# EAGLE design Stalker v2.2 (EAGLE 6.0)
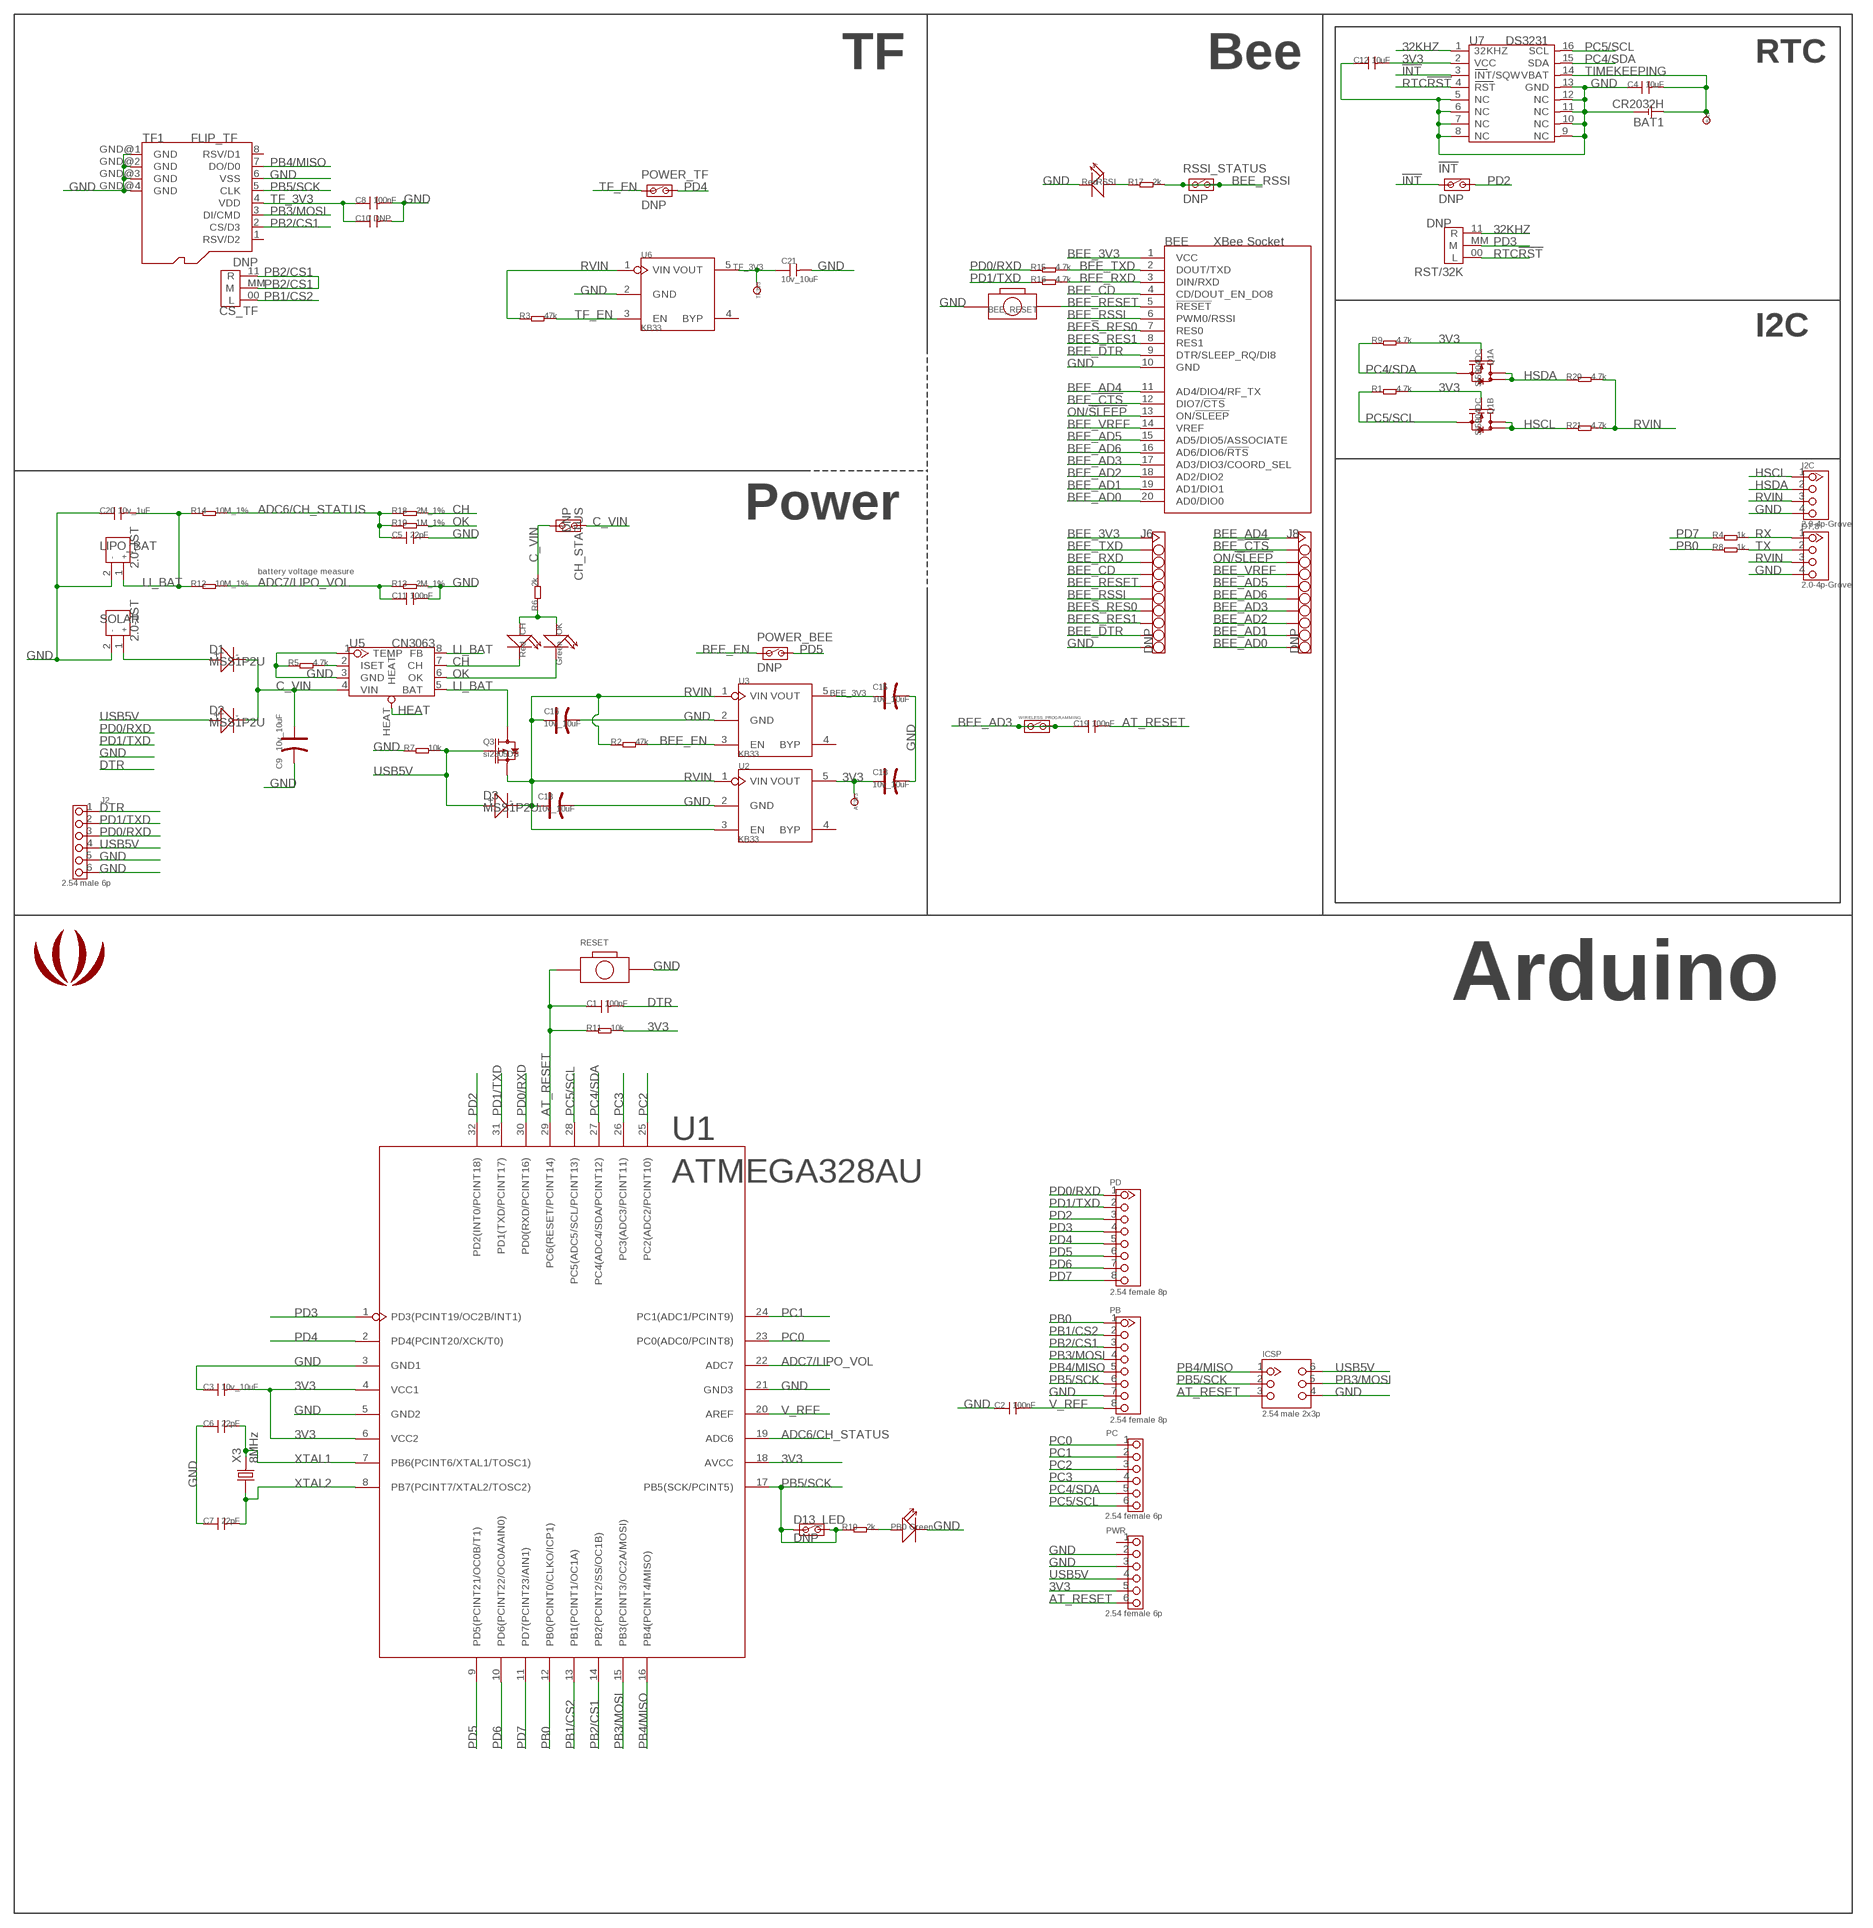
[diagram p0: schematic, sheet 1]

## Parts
!INT  DNP  JP_SW  [JP_SW]
AT3V3  DNP  TEST_POINT_SIZE_3030  [TP_3535]
BAT  DNP  TEST_POINT_SIZE_3030  [TP_3535]
BAT1  CR2032H  [CR2032H]
BEE  XBee Socket  BEEO  [BEE]
BEE_RESET  3.8x6.1 button  BOTTON_1_SMD  [BOTTON_1]
C1  100nF  C-0603  [0603]
C2  100nF  C-0603  [0603]
C3  10v_10uF  C-0805  [0805]
C4  10uF  C-0805  [0805]
C5  22pF  C-0603  [0603]
C6  22pF  C-0603  [0603]
C7  22pF  C-0603  [0603]
C8  100nF  C-0603  [0603]
C9  10v_10uF  CAP-AVX-A  [AVX-A]
C10  DNP  C-0603  [0603]
C11  100nF  C-0603  [0603]
C12  10uF  C-0805  [0805]
C13  10v_10uF  CAP-AVX-A  [AVX-A]
C15  10v_10uF  CAP-AVX-A  [AVX-A]
C16  10v_10uF  CAP-AVX-A  [AVX-A]
C18  10v_10uF  CAP-AVX-A  [AVX-A]
C19  100nF  C-0603  [0603]
C20  10v_1uF  C-0805  [0805]
C21  10v_10uF  C-0805  [0805]
CH  Red  007-LED0603  [D0603]
CH_STATUS  DNP  JP_SW  [JP_SW]
CS_TF  DNP  JUMPER  [JUMPER]
D1  MSS1P2U  010-DMSS1P2U  [D1005]
D2  MSS1P2U  010-DMSS1P2U  [D1005]
D3  MSS1P2U  010-DMSS1P2U  [D1005]
D7,8  2.0-4p-Grove  TWIG-4P-2.0-2.0  [4P-2.0]
D13_LED  DNP  JP_SW  [JP_SW]
I2C  2.0-4p-Grove  TWIG-4P-2.0-2.0  [4P-2.0]
ICSP  2.54 male 2x3p  HEADER-2X3P-2.54  [2X3P-2.54-LEADED]
J2  2.54 male 6p  HEADER-6P-LEADED-2.54  [6P-2.54-LEADED]
J6  DNP  HEADER_1X10DD  [HEADER_1X10]
J8  DNP  HEADER_1X10DD  [HEADER_1X10]
LIPO_BAT  2.0-JST  JACK-JST-2P-PW'2.0'  [JST-2.0]
LOGO1  LOGO  [LOGO_RO]
OK  Green  007-LED0603  [D0603]
PB  2.54 female 8p  HEADER-8P-2.54-LEADED  [8P-2.54-LEADED]
PB0  Green  007-LED0603  [D0603]
PC  2.54 female 6p  HEADER-6P-LEADED-2.54  [6P-2.54-LEADED]
PD  2.54 female 8p  HEADER-8P-2.54-LEADED  [8P-2.54-LEADED]
POWER_BEE  DNP  JP_SW  [JP_SW]
POWER_TF  DNP  JP_SW  [JP_SW]
PWR  2.54 female 6p  HEADER-6P-LEADED-2.54  [6P-2.54-LEADED]
Q1  Si5904DC  010-DUAL-N-MOSFET_1206-8  [1206-8]
Q3  si2305DS  010-P-MOSFETSOT23  [SOT23]
R1  4.7k  005-R0603  [0603@1]
R2  47k  005-R0603  [0603@1]
R3  47k  005-R0603  [0603@1]
R4  1k  005-R0603  [0603@1]
R5  4.7k  005-R0603  [0603@1]
R6  2k  005-R0603  [0603@1]
R7  10k  005-R0603  [0603@1]
R8  1k  005-R0603  [0603@1]
R9  4.7k  005-R0603  [0603@1]
R10  2k  005-R0603  [0603@1]
R11  10k  005-R0603  [0603@1]
R12  10M_1%  005-R0603  [0603@1]
R13  2M_1%  005-R0603  [0603@1]
R14  10M_1%  005-R0603  [0603@1]
R15  4.7k  005-R0603  [0603@1]
R16  4.7k  005-R0603  [0603@1]
R17  2k  005-R0603  [0603@1]
R18  2M_1%  005-R0603  [0603@1]
R19  1M_1%  005-R0603  [0603@1]
R20  4.7k  005-R0603  [0603@1]
R21  4.7k  005-R0603  [0603@1]
RESET  3.8x6.1 button  BOTTON_1_SMD  [BOTTON_1]
RSSI  Red  007-LED0603  [D0603]
RSSI_STATUS  DNP  JP_SW  [JP_SW]
RST/32K  DNP  JUMPER  [JUMPER]
SOLAR  2.0-JST  JACK-JST-2P-PW'2.0'  [JST-2.0]
TF1  FLIP_TF  [FLIP_TF]
TF3V3  DNP  TEST_POINT_SIZE_3030  [TP_3535]
U1  ATMEGA328AU  ATMEGA168-20AU  [ATMEGA168-20AU]
U2  KB33  MIC5025_X.X  [SOT23-5]
U3  KB33  MIC5025_X.X  [SOT23-5]
U5  CN3063  CN3083  [SOP8]
U6  KB33  MIC5025_X.X  [SOT23-5]
U7  DS3231  [SO16-W]
WIRELESS_PROGRAMMING  DNP  JP_SW  [JP_SW]
X3  8MHz  011-CRYSTALHC49S  [HC49/S]

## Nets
3V3: AT3V3.T C3.2 C12.2 C13.+ PWR.5 Q1.2(A:G) Q1.4(B:G) R1.2 R9.2 R11.2 U1.4(VCC1) U1.6(VCC2) U1.18(AVCC) U2.5(VOUT) U7.2(VCC)
32KHZ: RST/32K.11(R) U7.1(32KHZ)
!INT: !INT.1 U7.3(INT/SQW)
ADC6/CH_STATUS: C5.1 R14.2 R18.1 R19.1 U1.19(ADC6)
ADC7/LIPO_VOL: C11.1 R12.2 R13.1 U1.22(ADC7)
AT_RESET: C1.1 C19.2 ICSP.3 PWR.6 R11.1 RESET.1 U1.29(PC6(RESET/PCINT14))
BEE_3V3: BEE.1(VCC) C15.+ J6.1 U3.5(VOUT)
BEE_!CTS: BEE.12(DIO7/!CTS) J8.2
BEE_AD0: BEE.20(AD0/DIO0) J8.10
BEE_AD1: BEE.19(AD1/DIO1) J8.9
BEE_AD2: BEE.18(AD2/DIO2) J8.8
BEE_AD3: BEE.17(AD3/DIO3/COORD_SEL) C19.1 J8.7 WIRELESS_PROGRAMMING.1 WIRELESS_PROGRAMMING.2
BEE_AD4: BEE.11(AD4/DIO4/RF_TX) J8.1
BEE_AD5: BEE.15(AD5/DIO5/ASSOCIATE) J8.5
BEE_AD6: BEE.16(AD6/DIO6/!RTS) J8.6
BEE_CD: BEE.4(CD/DOUT_EN_DO8) J6.4
BEE_DTR: BEE.9(DTR/SLEEP_RQ/DI8) J6.9
BEE_EN: POWER_BEE.1 R2.2 U3.3(EN)
BEE_RESET: BEE.5(!RESET) BEE_RESET.P$2 J6.5
BEE_RSSI: BEE.6(PWM0/RSSI) J6.6 R17.2 RSSI_STATUS.1 RSSI_STATUS.2
BEE_RXD: BEE.3(DIN/RXD) J6.3 R16.2
BEE_TXD: BEE.2(DOUT/TXD) J6.2 R15.2
BEE_VREF: BEE.14(VREF) J8.4
BEES_RES0: BEE.7(RES0) J6.7
BEES_RES1: BEE.8(RES1) J6.8
C_VIN: C9.+ CH_STATUS.1 CH_STATUS.2 D1.- D2.- R6.2 U5.4(VIN)
CH: CH.- R18.2 U5.7(CH)
DTR: C1.2 J2.1
GND: BAT1.- BEE.10(GND) BEE_RESET.1 C2.1 C3.1 C4.1 C5.2 C6.1 C7.1 C8.2 C9.- C10.2 C11.2 C12.1 C13.- C15.- C16.- C18.- C20.1 C21.2 D7,8.4 I2C.4 ICSP.4 J2.5 J2.6 J6.10 LIPO_BAT.2 PB0.- PB.7 PWR.2 PWR.3 R5.1 R7.1 R13.2 RESET.P$2 RSSI.- SOLAR.2 TF1.6(VSS) TF1.GND@1(GND) TF1.GND@2(GND) TF1.GND@3(GND) TF1.GND@4(GND) U1.3(GND1) U1.5(GND2) U1.21(GND3) U2.2(GND) U3.2(GND) U5.1(TEMP) U5.3(GND) U6.2(GND) U7.5(NC) U7.6(NC) U7.7(NC) U7.8(NC) U7.9(NC) U7.10(NC) U7.11(NC) U7.12(NC) U7.13(GND)
HEAT: U5.HEAT
HSCL: I2C.1 Q1.5(B:D) Q1.6(B:D) R21.1
HSDA: I2C.2 Q1.7(A:D) Q1.8(A:D) R20.1
LI_BAT: C20.2 LIPO_BAT.1 Q3.3(D) R12.1 R14.1 U5.5(BAT) U5.8(FB)
N$1: PB0.+ R10.2
N$3: D1.+ SOLAR.1
N$5: R5.2 U5.2(ISET)
N$6: R17.1 RSSI.+
N$8: CH.+ OK.+ R6.1
OK: OK.- R19.2 U5.6(OK)
ON/!SLEEP: BEE.13(ON/!SLEEP) J8.3
PB0: PB.1 R8.1 U1.12(PB0(PCINT0/CLKO/ICP1))
PB1/CS2: CS_TF.00(L) PB.2 U1.13(PB1(PCINT1/OC1A))
PB2/CS1: CS_TF.11(R) CS_TF.MM(M) PB.3 TF1.2(CS/D3) U1.14(PB2(PCINT2/SS/OC1B))
PB3/MOSI: ICSP.5 PB.4 TF1.3(DI/CMD) U1.15(PB3(PCINT3/OC2A/MOSI))
PB4/MISO: ICSP.1 PB.5 TF1.7(DO/D0) U1.16(PB4(PCINT4/MISO))
PB5/SCK: D13_LED.1 D13_LED.2 ICSP.2 PB.6 R10.1 TF1.5(CLK) U1.17(PB5(SCK/PCINT5))
PC0: PC.1 U1.23(PC0(ADC0/PCINT8))
PC1: PC.2 U1.24(PC1(ADC1/PCINT9))
PC2: PC.3 U1.25(PC2(ADC2/PCINT10))
PC3: PC.4 U1.26(PC3(ADC3/PCINT11))
PC4/SDA: PC.5 Q1.1(A:S) R9.1 U1.27(PC4(ADC4/SDA/PCINT12)) U7.15(SDA)
PC5/SCL: PC.6 Q1.3(B:S) R1.1 U1.28(PC5(ADC5/SCL/PCINT13)) U7.16(SCL)
PD0/RXD: J2.3 PD.1 R15.1 U1.30(PD0(RXD/PCINT16))
PD1/TXD: J2.2 PD.2 R16.1 U1.31(PD1(TXD/PCINT17))
PD2: !INT.2 PD.3 U1.32(PD2(INT0/PCINT18))
PD3: PD.4 RST/32K.MM(M) U1.1(PD3(PCINT19/OC2B/INT1))
PD4: PD.5 POWER_TF.2 U1.2(PD4(PCINT20/XCK/T0))
PD5: PD.6 POWER_BEE.2 U1.9(PD5(PCINT21/OC0B/T1))
PD6: PD.7 U1.10(PD6(PCINT22/OC0A/AIN0))
PD7: PD.8 R4.1 U1.11(PD7(PCINT23/AIN1))
RTC!RST: RST/32K.00(L) U7.4(RST)
RVIN: C16.+ C18.+ D3.- D7,8.3 I2C.3 Q3.2(S) R2.1 R3.1 R20.2 R21.2 U2.1(VIN) U2.3(EN) U3.1(VIN) U6.1(VIN)
RX: D7,8.1 R4.2
TF_3V3: C8.1 C10.1 C21.1 TF1.4(VDD) TF3V3.T U6.5(VOUT)
TF_EN: POWER_TF.1 R3.2 U6.3(EN)
TIMEKEEPING: BAT1.+ BAT.T C4.2 U7.14(VBAT)
TX: D7,8.2 R8.2
USB5V: D2.+ D3.+ ICSP.6 J2.4 PWR.4 Q3.1(G) R7.2
V_REF: C2.2 PB.8 U1.20(AREF)
XTAL1: C6.2 U1.7(PB6(PCINT6/XTAL1/TOSC1)) X3.2
XTAL2: C7.2 U1.8(PB7(PCINT7/XTAL2/TOSC2)) X3.1
Unconnected: PWR.1 TF1.1(RSV/D2) TF1.8(RSV/D1) U2.4(BYP) U3.4(BYP) U6.4(BYP)

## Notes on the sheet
- TF | Bee | RTC
- I2C
- Power
- battery voltage measure
- Arduino

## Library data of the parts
!INT CH_STATUS D13_LED POWER_BEE POWER_TF RSSI_STATUS WIRELESS_PROGRAMMING = CPT_SMD:JP_SW
AT3V3 BAT TF3V3 = For_Test_Albert:TEST_POINT
BAT1 = BAT:CR2032H
BEE = EXT_moudle:BEE
BEE_RESET RESET = CPT_SMD:BOTTON_1
C1-C8 C10-C12 C19-C21 = Discrete:C*: Ceramic Capacitors
C9 C13 C15 C16 C18 = Discrete:CAP*: Electrolytic Capacitors,Tantalum Capacitors and Super Capacitors
CH OK PB0 RSSI = Discrete:007-LED*
CS_TF RST/32K = CPT_SMD:JUMPER
D1-D3 = Discrete:010-D*
D7,8 I2C = Connector:TWIG-4P-2.0
ICSP = Connector:HEADER-2X3P
J2 PC PWR = Connector:HEADER-6P
J6 J8 = CONNECTER:HEADER_1X10
LIPO_BAT SOLAR = Connector:JACK-JST-2P-PW
LOGO1 = logo:LOGO
PB PD = Connector:HEADER-8P
Q1 = Discrete:010-DUAL-N-MOSFET*: Si5902BDC Si5904DC Si5908DC Si5920DC
Q3 = Discrete:010-P-MOSFET*: Si2305DS Si2323CDS
R1-R21 = Discrete:005-R*
TF1 = Holders:FLIP_TF: http://garden.seeedstudio.com/images/e/e4/Flip_TF_Holder.jpg
U1 = IC_SMD:ATMEGA168-20AU
U2 U3 U6 = ICs_v54:MIC5025_X.X
U5 = ICs_v54:CN3083
U7 = IC:DS3231: Extremely Accurate I2C-Integrated RTC/TCXO/Crystal http://pdfserv.maxim-ic.com/en/ds/DS3231.pdf
X3 = Discrete:011-CRYSTAL*: CRYSTAL

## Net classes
0 default: width 0.152 mm, drill 0.305 mm, clearance 0.152 mm

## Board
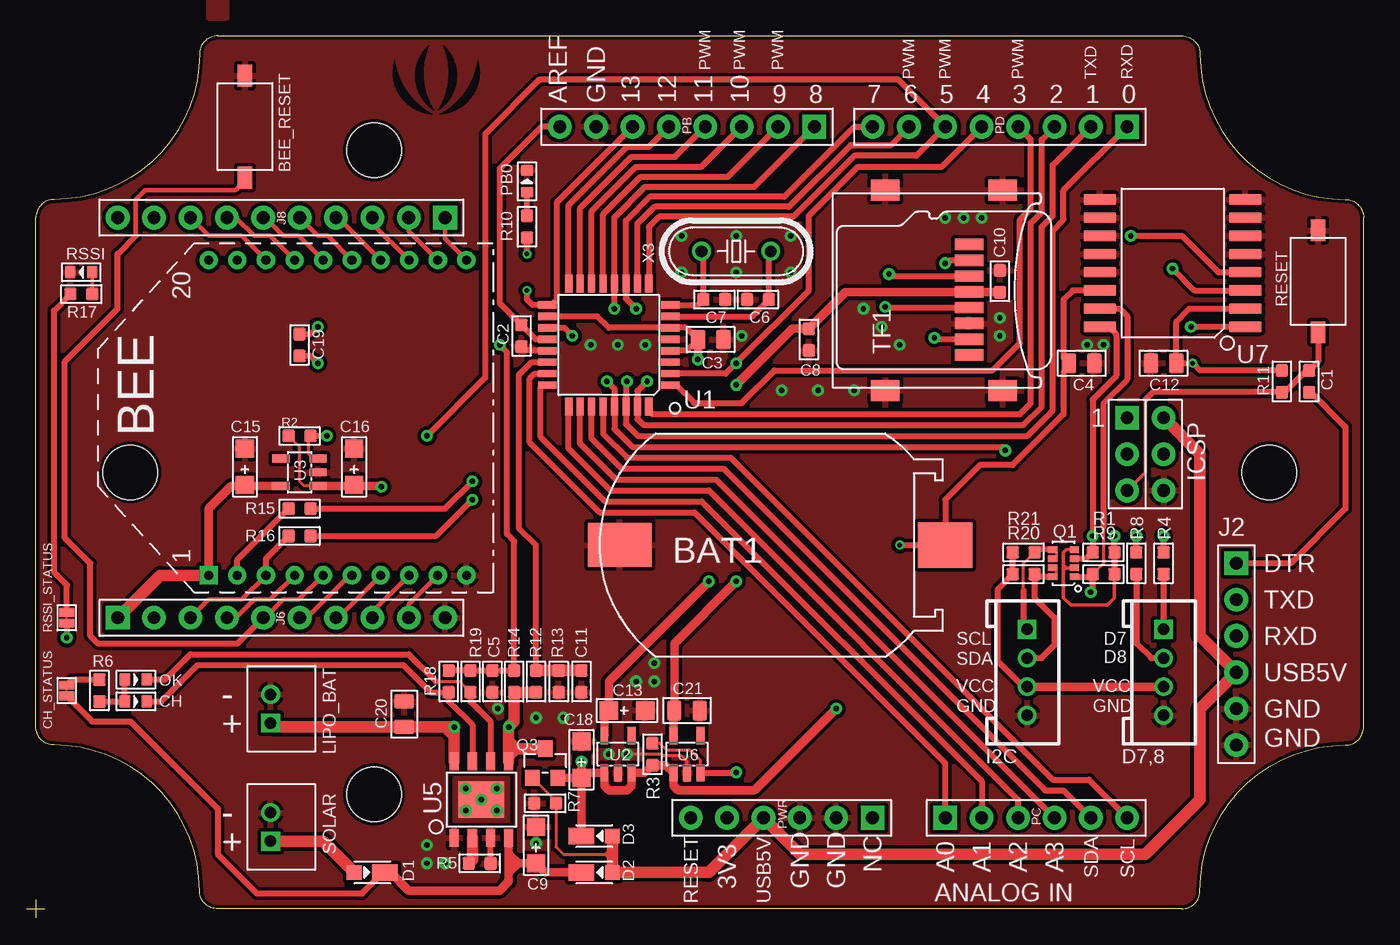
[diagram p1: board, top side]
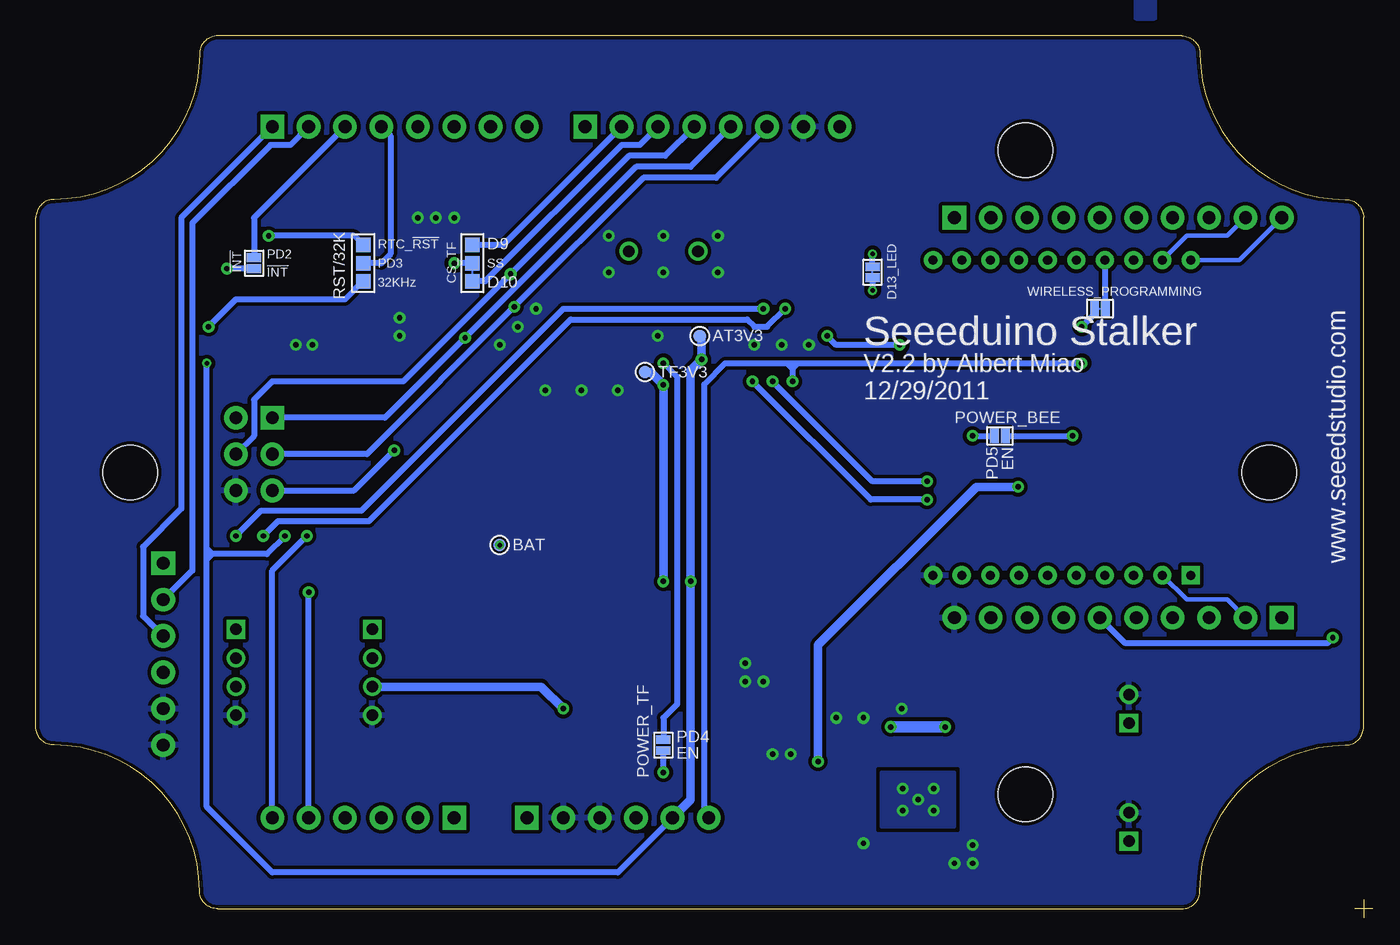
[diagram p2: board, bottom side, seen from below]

Size 92.71 x 60.96 mm. Coordinates in mm from the lower left corner, seen from the top.
Outline: 12.7,60.96 arc90 11.43,59.69 arc-90 1.27,49.53 arc90 0,48.26 0,12.7 arc90 1.27,11.43 arc-90 11.43,1.27 arc90 12.7,0 80.01,0 arc90 81.28,1.27 arc-90 91.44,11.43 arc90 92.71,12.7 92.71,48.26 arc90 91.44,49.53 arc-90 81.28,59.69 arc90 80.01,60.96 12.7,60.96
Copper layers (1*16): Top 0.035mm / dielectric 1.5mm / Bottom 0.035mm
Design rules: minimum track width 6mil, minimum drill 12mil, track to track 6mil, track to pad 6mil, pad to pad 6mil, via to via 6mil, smd to smd 0mil, copper to edge 10mil, drill to drill 10mil, minimum pad ring 10mil, minimum via ring 6mil, stop-mask expansion 2mil, vias tented up to drill 25mil, thermal gap 10mil
Holes 3.81 mm at 23.61,52.98 86.11,30.48 6.61,30.48 23.61,7.98
tRestrict: area 73.7,43.2 to 74.9,48.9; area 83.8,43.2 to 85.1,48.9
Milling: 2 lines

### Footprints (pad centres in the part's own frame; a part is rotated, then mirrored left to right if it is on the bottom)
JP_SW = smd 1.016 x 0.61: 1 0,0.381; 2 0,-0.381
TP_3535 = smd 0.889 x 0.889: T 0,0
CR2032H = smd 3.81 x 3.175: + 12.7,0 | smd 4.445 x 3.048: - -10.033,0
BEE = drill 0.635 pad 1.27 square: 1 -11,0 | drill 0.635 pad 1.27: 2 -11,-2; 3 -11,-4; 4 -11,-6; 5 -11,-8; 6 -11,-10; 7 -11,-12; 8 -11,-14; 9 -11,-16; 10 -11,-18; 11 11,-18; 12 11,-16; 13 11,-14; 14 11,-12; 15 11,-10; 16 11,-8; 17 11,-6; 18 11,-4; 19 11,-2; 20 11,0
BOTTON_1 = smd 1.524 x 1.016: 1 -3.556,0; P$2 3.556,0
0603 = smd 0.889 x 0.889: 1 -0.762,0; 2 0.762,0
0805 = smd 1.016 x 1.397: 1 -0.889,0; 2 0.889,0
AVX-A = smd 1.27 x 1.27: + -1.27,0; - 1.27,0
D0603 = smd 0.762 x 0.889: + -0.762,0; - 0.762,0
JUMPER = smd 1.016 x 1.016: 00 -1.27,0; 11 1.27,0; MM 0,0
D1005 = smd 1.016 x 1.016: + 1.27,0 | smd 1.778 x 1.143: - -0.889,0
4P-2.0 = drill 0.8 pad 1.27 square: 1 -3,0 | drill 0.8 pad 1.27: 2 -1,0; 3 1,0; 4 3,0
2X3P-2.54-LEADED = drill 0.889 pad 1.651 square: 1 -1.27,2.54 | drill 0.889 pad 1.651: 2 -1.27,0; 3 -1.27,-2.54; 4 1.27,-2.54; 5 1.27,0; 6 1.27,2.54
6P-2.54-LEADED = drill 0.889 pad 1.651 square: 1 0,6.35 | drill 0.889 pad 1.651: 2 0,3.81; 3 0,1.27; 4 0,-1.27; 5 0,-3.81; 6 0,-6.35
HEADER_1X10 = drill 0.889 pad 1.651 square: 1 0,11.43 | drill 0.889 pad 1.651: 2 0,8.89; 3 0,6.35; 4 0,3.81; 5 0,1.27; 6 0,-1.27; 7 0,-3.81; 8 0,-6.35; 9 0,-8.89; 10 0,-11.43
JST-2.0 = drill 0.8 pad 1.3 square: 1 -1,0.75 | drill 0.8 pad 1.3: 2 1,0.75
8P-2.54-LEADED = drill 0.889 pad 1.651 square: 1 0,8.89 | drill 0.889 pad 1.651: 2 0,6.35; 3 0,3.81; 4 0,1.27; 5 0,-1.27; 6 0,-3.81; 7 0,-6.35; 8 0,-8.89
1206-8 = smd 0.457 x 0.635: 1 -0.953,-0.762; 2 -0.318,-0.762; 3 0.318,-0.762; 4 0.953,-0.762; 5 0.953,0.762; 6 0.318,0.762; 7 -0.318,0.762; 8 -0.953,0.762
SOT23@1 = smd 1.016 x 1.143: 1 -0.889,-1.016; 2 0.889,-1.016; 3 0,1.016
0603@1 = smd 0.889 x 0.889: 1 -0.762,0; 2 0.762,0
FLIP_TF = smd 0.8 x 2: 1 3.2,0.25; 2 2.1,0.25; 3 1,0.25; 4 -0.1,0.25; 5 -1.2,0.25; 6 -2.3,0.25; 7 -3.4,0.25; 8 -4.5,0.25 | smd 1.45 x 2: GND@1 -7,6.1; GND@2 -7,-2.1; GND@3 7,-2.1; GND@4 7,6.1
ATMEGA168-20AU = smd 1.27 x 0.508: 1 -4.293,2.8; 2 -4.293,2; 3 -4.293,1.2; 4 -4.293,0.4; 5 -4.293,-0.4; 6 -4.293,-1.2; 7 -4.293,-2; 8 -4.293,-2.8; 17 4.293,-2.8; 18 4.293,-2; 19 4.293,-1.2; 20 4.293,-0.4; 21 4.293,0.4; 22 4.293,1.2; 23 4.293,2; 24 4.293,2.8 | smd 0.508 x 1.27: 9 -2.8,-4.293; 10 -2,-4.293; 11 -1.2,-4.293; 12 -0.4,-4.293; 13 0.4,-4.293; 14 1.2,-4.293; 15 2,-4.293; 16 2.8,-4.293; 25 2.8,4.293; 26 2,4.293; 27 1.2,4.293; 28 0.4,4.293; 29 -0.4,4.293; 30 -1.2,4.293; 31 -2,4.293; 32 -2.8,4.293
SOT23-5 = smd 0.55 x 1.2: 1 -0.95,-1.3; 2 0,-1.3; 3 0.95,-1.3; 4 0.95,1.3; 5 -0.95,1.3
SOP8 = smd 0.635 x 1.27: 1 -1.905,-2.667; 2 -0.635,-2.667; 3 0.635,-2.667; 4 1.905,-2.667; 5 1.905,2.667; 6 0.635,2.667; 7 -0.635,2.667; 8 -1.905,2.667 | smd 3.175 x 2.54: HEAT 0,0
SO16-W = smd 0.762 x 2.286: 1 -4.445,-5.08; 2 -3.175,-5.08; 3 -1.905,-5.08; 4 -0.635,-5.08; 5 0.635,-5.08; 6 1.905,-5.08; 7 3.175,-5.08; 8 4.445,-5.08; 9 4.445,5.08; 10 3.175,5.08; 11 1.905,5.08; 12 0.635,5.08; 13 -0.635,5.08; 14 -1.905,5.08; 15 -3.175,5.08; 16 -4.445,5.08
HC49/S = drill 0.813: 1 -2.413,0; 2 2.413,0

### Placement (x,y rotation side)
!INT  77.47,45.09 180 bottom
AT3V3  46.35,40.01 0 bottom
BAT  60.33,25.4 0 bottom
BAT1  50.8,25.4 0 top
BEE  12.06,34.29 90 top
BEE_RESET  14.61,54.61 270 top
C1  88.9,36.83 270 top
C2  33.91,40.01 90 top
C3  47.12,39.75 180 top
C4  73.03,38.1 180 top
C5  31.88,15.88 270 top
C6  50.42,42.55 0 top
C7  47.37,42.55 180 top
C8  53.98,39.75 270 top
C9  34.92,4.45 90 top
C10  67.31,43.81 90 top
C11  38.1,15.88 270 top
C12  78.74,38.1 0 top
C13  41.27,13.84 0 top
C15  14.61,30.86 90 top
C16  22.23,30.86 90 top
C18  38.1,10.41 90 top
C19  18.41,39.37 270 top
C20  25.72,13.59 270 top
C21  45.47,13.84 0 top
CH  6.99,14.48 0 top
CH_STATUS  2.16,15.24 180 top
CS_TF  62.23,45.09 270 bottom
D1  23.5,2.54 180 top
D2  38.99,2.54 0 top
D3  38.99,5.08 0 top
D7,8  78.74,16.51 270 top
D13_LED  34.29,44.45 180 bottom
I2C  69.22,16.51 270 top
ICSP  77.47,31.75 0 top
J2  83.82,17.78 0 top
J6  17.14,20.32 90 top
J8  17.14,48.26 270 top
LIPO_BAT  17.14,13.97 90 top
LOGO1  27.94,57.15 0 top
OK  6.99,16 0 top
PB  45.47,54.61 270 top
PB0  34.29,50.8 90 top
PC  69.85,6.35 90 top
PD  67.31,54.61 270 top
POWER_BEE  25.4,33.02 270 bottom
POWER_TF  48.9,11.43 180 bottom
PWR  52.07,6.35 270 top
Q1  71.75,24.13 90 top
Q3  si2305DS  [SOT23@1]  35.56,10.16 0 top
R1  74.55,24.89 0 top
R2  18.41,33.02 0 top
R3  43.05,10.79 90 top
R4  78.74,24.13 270 top
R5  30.99,3.17 180 top
R6  4.45,15.24 90 top
R7  35.56,7.37 0 top
R8  76.83,24.13 270 top
R9  74.55,23.37 0 top
R10  34.29,47.62 90 top
R11  87,36.83 90 top
R12  34.92,15.88 90 top
R13  36.51,15.88 270 top
R14  33.4,15.88 90 top
R15  18.41,27.94 180 top
R16  18.41,26.04 180 top
R17  3.17,42.93 180 top
R18  28.83,15.88 270 top
R19  30.35,15.88 270 top
R20  68.96,23.37 180 top
R21  68.96,24.89 180 top
RESET  89.53,43.81 90 top
RSSI  3.17,44.45 180 top
RSSI_STATUS  2.16,20.32 0 top
RST/32K  69.85,45.09 270 bottom
SOLAR  17.14,5.71 90 top
TF1  65.41,43.18 90 top
TF3V3  50.16,37.47 0 bottom
U1  40.01,39.37 180 top
U2  40.64,10.79 0 top
U3  18.41,30.48 90 top
U5  31.11,7.62 0 top
U6  45.47,10.79 0 top
U7  79.38,45.09 90 top
WIRELESS_PROGRAMMING  18.41,41.91 270 bottom
X3  48.9,45.91 0 top

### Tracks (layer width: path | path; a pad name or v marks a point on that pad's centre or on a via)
3V3  (via drill 0.3 pad 0.64, 0.38 pad 0.81)
  Top 0.254: Q1.4 71.94,25.08 71.75,24.89 71.75,24 | Q1.2 71.94,23.81 | 71.94,23.81 71.75,24 | R9.2 75.31,21.72 74.8,21.21 72.26,21.21 71.75,21.72 71.75,23.62 | 71.75,23.62 71.75,24 | 71.94,23.81 71.75,23.62
  Top 0.406: U1.4 45.45,38.97 C3.2 45.41,40.57 U1.6 40.01,40.57 39.21,41.37 U1.18 | R11.2 81.28,37.59 v80.77,38.1 C12.2 79.63,41.02 80.52,41.91 U7.2 | R9.2 R1.2 v75.31,26.04
  Top 0.61: v46.23,38.35 C3.2 | U2.5 39.69,13.53 C13.+ 40.01,15.88 v46.99,22.86
  Bottom 0.406: PWR.5 52.07,2.54 76.2,2.54 80.77,7.11 80.77,24.38 | 80.77,24.38 80.77,25.15 | 80.77,25.15 v80.77,38.1 | v75.31,26.04 76.58,24.77 80.39,24.77 | 80.39,24.77 80.77,25.15 | 80.77,24.38 80.39,24.77
  Bottom 0.61: PWR.5 46.99,7.62 v46.99,22.86 46.99,37.59 v46.23,38.35 46.23,39.88 AT3V3.T
  pour Bottom: 14.61,63.5 15.88,63.5 15.88,62.23 14.61,62.23
32KHZ  (via drill 0.38 pad 0.81)
  Top 0.406: v80.64,40.64 U7.1
  Bottom 0.406: RST/32K.11 71.12,42.55 78.74,42.55 v80.64,40.64
!INT  (via drill 0.38 pad 0.81)
  Top 0.406: U7.3 80.9,43.18 v79.38,44.7
  Bottom 0.406: !INT.1 v79.38,44.7
ADC6/CH_STATUS  (via drill 0.38 pad 0.81)
  Top 0.406: R18.1 R19.1 C5.1 R14.2 33.4,25.65 32.89,26.16 32.89,38.86 v32.38,39.37 | U1.19 36.9,40.57 v37.47,40.01
  Bottom 0.406: v32.38,39.37 36.83,39.37 v37.47,40.01
ADC7/LIPO_VOL
  Top 0.406: U1.22 34.61,38.17 33.72,37.27 33.72,26.61 34.92,25.4 R12.2
  Top 0.813: R12.2 R13.1 C11.1
AT_RESET  (via drill 0.38 pad 0.81)
  Top 0.254: 77.47,35.56 77.47,30.48 ICSP.3
  Top 0.406: v39.88,36.83 40.41,36.3 U1.29 40.41,33.51 41.66,32.26 67.44,32.26 v67.69,32 | C19.2 19.18,38.61 v19.68,38.1 | 77.47,35.56 77.98,36.07 R11.1 87.19,36.07 88.71,37.59 C1.1 89.53,38.23 RESET.1
  Bottom 0.406: PWR.6 46.04,6.67 46.04,36.64 44.58,38.1 40.26,38.1 | 40.26,38.1 39.5,38.1 | 39.88,37.72 v39.88,36.83 | 39.5,38.1 39.88,37.72 | 40.26,38.1 39.88,37.72 | 39.5,38.1 v19.68,38.1 | ICSP.3 70.48,29.21 v67.69,32
BEE_3V3
  Top 0.61: U3.5 14.61,29.53 | 14.61,29.53 13.65,29.53 12.06,27.94 BEE.1 | C15.+ 14.61,29.53
  Top 0.813: BEE.1 8.69,23.29 J6.1
BEE_!CTS
  Top 0.305: BEE.12 26.04,47.32 J8.2
BEE_AD0
  Bottom 0.305: BEE.20 8.69,45.29 J8.10
BEE_AD1
  Bottom 0.305: BEE.19 12.37,46.99 9.53,46.99 J8.9
BEE_AD2
  Top 0.305: BEE.18 14.37,46.99 12.06,46.99 J8.8
BEE_AD3  (via drill 0.38 pad 0.81)
  Top 0.305: BEE.17 16.36,46.99 15.24,46.99 13.97,48.26 J8.7
  Top 0.406: C19.1 19.18,40.13 v19.68,40.64
  Bottom 0.152: WIRELESS_PROGRAMMING.2 WIRELESS_PROGRAMMING.1
  Bottom 0.406: WIRELESS_PROGRAMMING.1 18.03,45.26 BEE.17 | WIRELESS_PROGRAMMING.2 18.8,41.53 v19.68,40.64
BEE_AD4
  Top 0.305: BEE.11 28.57,46.78 J8.1
BEE_AD5
  Top 0.305: BEE.15 20.36,46.99 19.68,46.99 J8.5
BEE_AD6
  Top 0.305: BEE.16 18.36,46.99 17.27,46.99 16,48.26 J8.6
BEE_CD
  Top 0.305: BEE.4 16.36,21.59 15.24,21.59 13.97,20.32 J6.4
BEE_DTR
  Top 0.305: J6.9 26.04,21.26 BEE.9
BEE_EN  (via drill 0.38 pad 0.81)
  Top 0.203: U3.3 19.37,31.43 19.05,31.75 19.05,32.89 R2.2
  Top 0.406: v20.32,33.02 R2.2
  Bottom 0.406: POWER_BEE.1 v20.32,33.02
BEE_RESET
  Top 0.305: 6.99,46.99 6.99,49.53 7.62,50.16 13.97,50.16 14.61,50.8 BEE_RESET.P$2 | BEE.5 18.36,21.59 17.27,21.59 16,20.32 J6.5
  Top 0.406: J6.5 14.1,18.54 4.32,18.54 3.81,19.05 3.81,24.13 2.03,25.91 2.03,38.23 5.71,41.91 5.71,45.72 6.99,46.99
BEE_RSSI  (via drill 0.38 pad 0.81)
  Top 0.152: RSSI_STATUS.2 RSSI_STATUS.1
  Top 0.305: J6.6 18.92,20.32 21.89,23.29 BEE.6
  Top 0.406: R17.2 1.27,41.78 1.27,23.5 2.16,22.61 RSSI_STATUS.1 | RSSI_STATUS.2 v2.16,18.92
  Bottom 0.406: J6.6 16.64,18.54 2.54,18.54 v2.16,18.92
BEE_RXD
  Top 0.305: BEE.3 14.37,21.59 12.06,21.59 J6.3
  Top 0.406: BEE.3 16.07,24.45 R16.2
BEE_TXD
  Top 0.406: BEE.2 14.06,24.35 R15.2
  Bottom 0.305: BEE.2 12.37,21.59 9.53,21.59 J6.2
BEE_VREF
  Top 0.305: BEE.14 21.09,48.26 J8.4
BEES_RES0
  Top 0.305: J6.7 21.09,20.32 BEE.7
BEES_RES1
  Top 0.305: J6.8 23.5,20.72 BEE.8
C_VIN
  Top 0.152: CH_STATUS.1 CH_STATUS.2
  Top 0.406: D1.- 24.26,2.54 22.8,1.08 15.43,1.08 12.7,3.81 12.7,6.99 6.6,13.08 3.94,13.08 CH_STATUS.1 | R6.2 2.54,16 CH_STATUS.2
  Top 0.61: D1.- 24.77,2.54 26.04,1.27 32.38,1.27 33.02,1.91 33.02,2.54 | 33.02,2.54 33.02,3.17 | 33.02,3.17 33.02,3.81 | 33.02,3.81 U5.4 | 33.66,3.17 C9.+ 35.56,2.54 D2.- | 33.66,3.17 33.02,3.17 | 33.66,3.17 33.02,3.81 | 33.66,3.17 33.02,2.54
CH
  Top 0.406: CH.- 8.76,14.48 11.3,17.02 25.65,17.02 27.56,15.11 R18.2 28.83,14.48 30.48,12.83 U5.7
DTR
  Top 0.406: C1.2 89.03,36.07 91.44,33.66 91.44,27.94 87.63,24.13 J2.1
GND  (via drill 0.38 pad 0.81)
  Top 0.203: U6.2 45.47,10.29 45.09,10.67 43.81,10.67 43.69,10.79 v41.27,10.79
  Top 0.406: U1.21 34.18,38.97 C2.1 | R5.1 U5.3
  other vias: 73.41,39.37 74.55,39.37 67.31,41.27 67.31,40.01 57.78,41.91 59.05,40.64 60.33,39.37 66.04,48.26 64.77,48.26 63.5,48.26 57.15,36.2 54.61,36.2 52.07,36.2 49.28,40.01 38.73,39.37 40.64,39.37 42.55,39.37 45.09,44.45 45.09,46.99 48.9,46.99 48.9,44.45 52.7,44.45 52.7,46.99 32.26,13.97 34.92,13.34 36.83,13.34 41.91,15.88 43.18,15.88 43.18,17.14 40.01,10.79 28.57,3.17 27.3,3.17 27.3,4.45 34.92,4.57
  pour Top (rank 6): 13.34,63.5 12.06,63.5 12.06,62.23 13.34,62.23
  pour Top (rank 5, no thermals): 24.13,60.96 31.75,60.96 31.75,56.52 29.84,54.61 26.04,54.61 24.13,56.52
  pour Bottom (isolate 0.254, rank 6): 0,60.96 92.71,60.96 92.71,0 0,0
  pour Top (isolate 0.254, rank 6): 0,60.96 92.71,60.96 92.71,0 0,0
HEAT  (via drill 0.38 pad 0.81)
  other vias: 30.04,8.38 30.04,6.86 32.19,6.86 32.19,8.38 31.11,7.62
  pour Bottom (isolate 0.254): 28.57,9.53 33.66,9.53 33.66,5.71 28.57,5.71
  pour Top (isolate 0.254, no thermals): 29.21,9.14 33.02,9.14 33.02,6.1 29.21,6.1
HSCL
  Top 0.203: Q1.6 71.06,24.45 71.25,24.64 71.25,24.89 71.06,25.08 Q1.5 | 68.96,22.23 68.96,24.13 R21.1
  Top 0.406: Q1.5 69.91,25.08 R21.1 | 68.96,22.23 68.96,19.76 I2C.1
HSDA
  Top 0.203: Q1.7 71.06,23.81 71.25,23.62 71.25,23.37 71.06,23.18 Q1.8
  Top 0.406: Q1.8 69.91,23.18 R20.1 69.72,21.72 71.12,20.32 71.12,18.41 70.22,17.51 I2C.2
LI_BAT  (via drill 0.38 pad 0.81)
  Top 0.813: v29.21,12.7 C20.2 16.66,12.7 LIPO_BAT.1 | 33.02,11.68 v33.02,12.7 33.4,13.08 R14.1 R12.1 | 33.02,11.68 33.02,10.67 | 33.02,10.67 U5.5 | v29.21,12.7 28.57,12.7 29.21,12.06 v29.21,12.7 | v29.21,12.7 U5.8 | 33.53,11.18 Q3.3 | 33.02,11.68 33.53,11.18 | 33.02,10.67 33.53,11.18
  Bottom 0.813: v29.21,12.7 v33.02,12.7
N$1
  Top 0.406: R10.2 PB0.+
N$3
  Top 0.813: D1.+ 20.05,4.71 SOLAR.1
N$5
  Top 0.813: U5.2 30.48,3.43 R5.2
N$6
  Top 0.254: R17.1 RSSI.+
N$8
  Top 0.406: R6.1 CH.+ OK.+
OK
  Top 0.203: 27.94,15.88 29.59,15.88 R19.2
  Top 0.406: OK.- 9.02,16 10.79,17.78 26.04,17.78 27.94,15.88 | U5.6 31.75,13.08 30.35,14.48 R19.2
ON/!SLEEP
  Top 0.305: BEE.13 23.5,47.86 J8.3
PB0  (via drill 0.38 pad 0.81)
  Top 0.406: PB.1 50.16,50.42 42.55,50.42 40.41,48.28 U1.12 40.41,41.93 v40.39,41.91 | R8.1 v76.83,26.04
  Bottom 0.406: v40.39,41.91 41.66,40.64 42.55,40.64 43.05,41.15 55.37,41.15 69.47,27.05 75.82,27.05 v76.83,26.04
PB1/CS2
  Top 0.406: U1.13 39.6,48.49 42.23,51.12 48.32,51.12 PB.2
  Bottom 0.406: CS_TF.00 60.07,46.35 PB.2
PB2/CS1  (via drill 0.38 pad 0.81)
  Top 0.406: U1.14 38.8,48.71 41.91,51.82 46.48,51.82 PB.3 | TF1.2 63.7,45.28 v63.5,45.09
  Bottom 0.152: CS_TF.11 CS_TF.MM
  Bottom 0.406: CS_TF.MM v63.5,45.09 | PB.3 50.55,53.34 51.82,53.34 61.34,43.81 CS_TF.11
PB3/MOSI  (via drill 0.38 pad 0.81)
  Top 0.406: U1.15 38.01,48.93 41.59,52.51 44.64,52.51 PB.4 | TF1.3 59.71,44.18 v59.56,44.32
  Bottom 0.406: PB.4 48.77,52.58 51.31,52.58 v59.56,44.32 67.06,36.83 76.2,36.83 77.47,35.56 77.47,33.02 ICSP.5
PB4/MISO  (via drill 0.38 pad 0.81)
  Top 0.406: U1.16 37.2,49.14 41.27,53.21 42.8,53.21 PB.5 | TF1.7 62.84,39.78 v62.74,39.88
  Bottom 0.406: PB.5 46.99,51.82 50.8,51.82 v62.74,39.88 68.33,34.29 ICSP.1
PB5/SCK  (via drill 0.3 pad 0.64, 0.38 pad 0.81)
  Top 0.406: PB.6 36.39,49.34 36.39,42.55 36.01,42.17 U1.17 34.66,42.17 34.29,42.55 v34.29,43.18 | TF1.5 59.37,41.98 v59.31,42.04 | v34.29,45.72 R10.1
  Bottom 0.152: D13_LED.1 D13_LED.2
  Bottom 0.406: PB.6 45.21,51.05 50.29,51.05 v59.31,42.04 69.6,31.75 ICSP.2 | D13_LED.2 v34.29,45.72 | D13_LED.1 v34.29,43.18
PC0
  Top 0.406: U1.23 34.83,37.37 34.48,37.02 34.48,32.58 39.37,27.69 45.97,27.69 63.5,10.16 PC.1
PC1
  Top 0.406: U1.24 35.36,36.57 35.24,36.45 35.24,32.96 39.75,28.45 46.48,28.45 66.04,8.89 PC.2
PC2
  Top 0.406: U1.25 37.2,32.14 40.13,29.21 46.99,29.21 68.58,7.62 PC.3
PC3
  Top 0.406: U1.26 38.01,32.48 40.51,29.97 47.5,29.97 PC.4
PC4/SDA  (via drill 0.38 pad 0.81)
  Top 0.203: 74.55,26.67 74.55,24.13 R9.1
  Top 0.406: U1.27 38.8,32.82 40.89,30.73 48.01,30.73 70.48,8.26 71.75,8.26 PC.5 | U7.15 75.69,41.91 76.2,41.4 76.2,36.96 74.55,35.31 74.55,26.67 | Q1.1 73.6,23.18 R9.1 73.79,22.23 v73.66,22.1
  Bottom 0.406: PC.5 v73.66,22.1
PC5/SCL  (via drill 0.38 pad 0.81)
  Top 0.406: U1.28 39.6,33.17 41.27,31.5 48.51,31.5 70.99,9.02 73.53,9.02 PC.6 | U7.16 74.93,40.64 75.44,40.13 75.44,37.21 73.79,35.56 v73.79,26.04 R1.1 73.34,24.45 Q1.3
  Bottom 0.406: PC.6 76.2,23.62 v73.79,26.04
PD0/RXD  (via drill 0.38 pad 0.81)
  Top 0.406: v41.27,36.83 41.2,36.76 U1.30 41.2,33.85 42.04,33.02 69.22,33.02 70.99,34.8 70.99,47.37 71.75,48.13 71.75,50.16 PD.1 | R15.1 28.57,27.94 v30.48,29.84
  Bottom 0.406: PD.1 82.55,48.26 82.55,27.94 85.22,25.27 85.22,20.45 J2.3 | v30.48,29.84 34.29,29.84 v41.27,36.83
PD1/TXD  (via drill 0.38 pad 0.81)
  Top 0.406: v42.67,36.83 42.01,36.16 U1.31 42.01,34.2 42.42,33.78 68.96,33.78 70.23,35.05 70.23,47.62 70.99,48.39 70.99,51.94 PD.2 | R16.1 27.94,26.04 v30.48,28.57
  Bottom 0.406: PD.2 74.93,53.34 76.33,53.34 81.79,47.88 81.79,23.62 J2.2 | v30.48,28.57 34.42,28.57 v42.67,36.83
PD2
  Top 0.406: PD.3 70.23,53.72 70.23,48.64 69.47,47.88 69.47,35.31 68.71,34.54 43.05,34.54 42.8,34.79 U1.32
  Bottom 0.406: !INT.2 77.47,48.26 PD.3
PD3
  Top 0.406: U1.1 44.71,36.57 45.97,35.31 49.28,35.31 51.56,37.59 66.8,37.59 68.71,39.5 68.71,48.13 69.47,48.9 69.47,53.72 PD.4
  Bottom 0.406: RST/32K.MM 68.58,45.09 67.94,45.72 67.94,53.98 PD.4
PD4  (via drill 0.38 pad 0.81)
  Top 0.406: U1.2 48.16,37.37 v48.9,38.1 53.98,43.18 53.98,48.39 57.4,51.82 63.25,51.82 PD.5
  Bottom 0.406: v48.9,38.1 47.94,37.15 47.94,14.29 48.9,13.34 POWER_TF.2
PD5  (via drill 0.38 pad 0.81)
  Top 0.406: U1.9 42.8,47.63 43.5,48.32 52.9,48.32 57.15,52.58 61.47,52.58 PD.6 60.2,57.91 35.18,57.91 31.37,54.1 31.37,37.08 v27.3,33.02
  Bottom 0.406: v27.3,33.02 POWER_BEE.2
PD6
  Top 0.406: U1.10 42.01,47.85 43.18,49.02 52.58,49.02 56.9,53.34 59.69,53.34 PD.7
PD7  (via drill 0.38 pad 0.81)
  Top 0.406: PD.8 57.15,54.61 52.26,49.72 42.86,49.72 41.2,48.06 U1.11 41.2,42.62 v41.91,41.91 | R4.1 v78.74,26.04
  Bottom 0.406: v78.74,26.04 76.96,27.81 69.98,27.81 55.88,41.91 v41.91,41.91
RTC!RST  (via drill 0.38 pad 0.81)
  Top 0.406: U7.4 82.55,44.45 80.01,46.99 v76.45,46.99
  Bottom 0.406: v76.45,46.99 70.48,46.99 RST/32K.00
RVIN  (via drill 0.38 pad 0.81)
  Top 0.203: U3.1 18.73,29.53 18.41,29.84 18.41,32.26 R2.1
  Top 0.406: R21.2 R20.2 67.18,22.35 67.18,17.27 68.94,15.51 I2C.3
  Top 0.61: D3.- C18.+ | Q3.2 C18.+ | U3.1 22.16,29.53 | 22.16,29.53 C16.+ | 22.16,29.53 24.06,29.53 v24.13,29.46 | v38.1,10.29 C18.+ | C18.+ 38.45,9.49 U2.1 39.69,8.57 40.01,8.26 41.27,8.26 41.59,8.57 U2.3 42.52,9.49 R3.1 43.98,10.03 U6.1 44.52,8.57 44.83,8.26 50.16,8.26 v55.88,13.97 | I2C.3 D7,8.3
  Bottom 0.61: v24.13,29.46 27.05,29.46 38.1,18.41 v38.1,10.29 | v55.88,13.97 57.42,15.51 I2C.3
RX
  Top 0.406: D7,8.1 R4.2
TF_3V3  (via drill 0.38 pad 0.81)
  Top 0.61: C10.1 67.28,43.08 TF1.4 56.54,43.08 C8.1 52.83,40.51 v48.9,36.58 | U6.5 44.52,13.78 C21.1 44.58,18.54 v48.9,22.86
  Bottom 0.61: v48.9,22.86 v48.9,36.58 49.78,37.47 TF3V3.T
TF_EN  (via drill 0.38 pad 0.81)
  Top 0.203: U6.3 46.42,10.35 45.72,11.05 44.07,11.05 43.56,11.56 R3.2
  Top 0.406: U6.3 48.87,9.49 v48.9,9.53
  Bottom 0.406: v48.9,9.53 POWER_TF.1
TIMEKEEPING  (via drill 0.3 pad 0.64)
  Top 0.406: BAT.T BAT1.+ 63.5,28.57 65.91,30.99 68.2,30.99 71.75,34.54 71.75,37.47 72.14,37.85 C4.2 71.75,38.48 71.75,42.55 72.39,43.18 U7.14
  other vias: 60.33,25.4
TX
  Top 0.406: R8.2 76.83,18.54 77.87,17.51 D7,8.2
USB5V
  Top 0.203: Q3.1 36.32,7.49 R7.2 36.32,4.32 36.83,3.81 39.75,3.81 | 39.75,3.81 40.26,4.32 | 40.26,3.3 39.75,3.81
  Top 0.813: D3.+ 40.26,4.32 40.26,3.3 D2.+ 46.99,2.54 PWR.4 53.34,3.81 77.47,3.81 81.28,7.62 81.28,13.97 J2.4 81.28,19.05 81.28,31.75 ICSP.6
V_REF
  Top 0.406: U1.20 34.91,39.77 C2.2 32.38,42.29 32.38,51.69 35.31,54.61 PB.8
XTAL1
  Top 0.406: U1.7 50.01,41.37 C6.2 51.18,45.78 X3.2
XTAL2
  Top 0.406: U1.8 46.23,42.17 C7.2 46.61,45.78 X3.1

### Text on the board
tPlace: PWM | PWM | PWM | PWM | PWM | PWM | TXD | RXD | AREF | GND | 13 | 12 | 11 | 10 | 9 | 8 | 7 | 6 | 5 | 4 | 3 | 2 | 1 | 0 | 1 | DTR | TXD | SCL | D7 | RXD | SDA | D8 | USB5V | VCC | VCC | - | GND | GND | GND | + | GND | - | + | NC | A0 | A1 | A2 | A3 | SDA | SCL | 3V3 | GND | GND | ANALOG IN | RESET | USB5V
bPlace: D9 | RTC_!RST | SS | PD3 | PD2 | !INT | D10 | 32KHz | Seeeduino Stalker | V2.2 by Albert Miao | 12/29/2011 | EN | PD5 | www.seeedstudio.com | PD4 | EN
